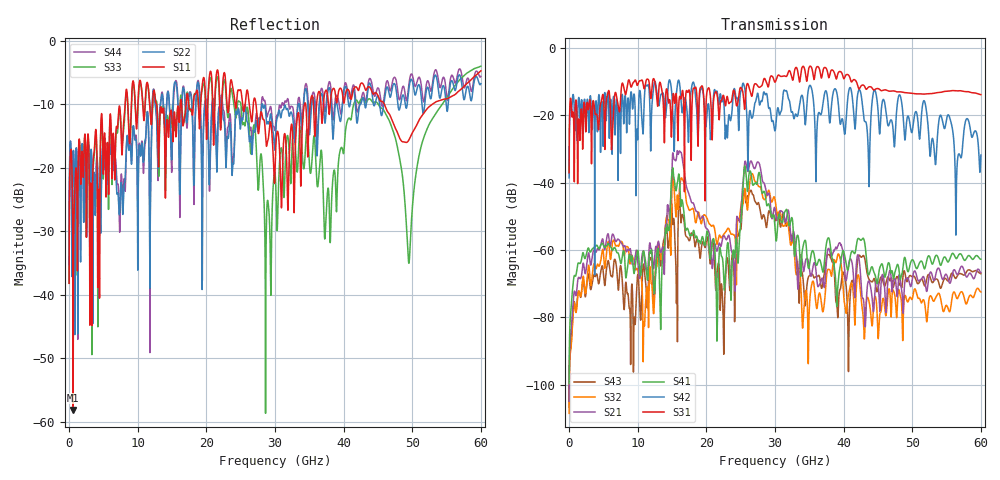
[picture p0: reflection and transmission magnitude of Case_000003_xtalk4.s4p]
! Info: Touchstone file created by circ.  Input file=CasetestDOE_NRZ_template_000003.circ
# Hz S RI R 50
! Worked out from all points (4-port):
!   6000 points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, 10 MHz to 60 GHz, reference 50 ohm
!   strongest paths, dB at 10 MHz, 15.01 GHz, 30.01 GHz, 45.01 GHz, 60 GHz:
!     S31: -37.0, -19.6, -10.2, -12.0, -13.8
!     S42: -38.6, -14.8, -24.6, -18.3, -31.8
!     S41: -99.6, -36.8, -53.6, -68.8, -62.7
!     S21: -104.9, -34.9, -47.7, -69.8, -66.7
!     S32: -108.5, -40.8, -45.0, -85.6, -72.4
!     S43: -106.7, -48.1, -50.8, -71.3, -67.0
!   lowest |S11| = -58.2 dB at 600 MHz (marker M1), VSWR 1.00, Z = 49.9 - j0.0876 ohm
!   |S11| at or under -10 dB: start of sweep to 8.166 GHz; 27.23 GHz to 34.3 GHz (7.064 GHz wide, 23 % of centre); 45.92 GHz to 52.96 GHz (7.036 GHz wide, 14.2 % of centre)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
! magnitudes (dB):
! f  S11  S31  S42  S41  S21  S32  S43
! 10 MHz  -38.2  -37.0  -38.6  -99.6  -104.9  -108.5  -106.7
! 600 MHz  -58.2  -19.1  -13.8  -69.8  -75.1  -78.8  -78.1
! 16.03 GHz  -12.7  -15.5  -9.8  -37.6  -30.8  -43.9  -45.0
! 21.57 GHz  -4.7  -13.9  -12.9  -85.5  -60.3  -58.3  -66.8
! 25.63 GHz  -10.3  -17.3  -12.4  -35.1  -33.7  -41.8  -42.9
! 49.5 GHz  -15.7  -13.4  -20.7  -66.0  -69.0  -74.8  -68.0
! 60 GHz  -4.8  -13.8  -31.8  -62.7  -66.7  -72.4  -67.0
